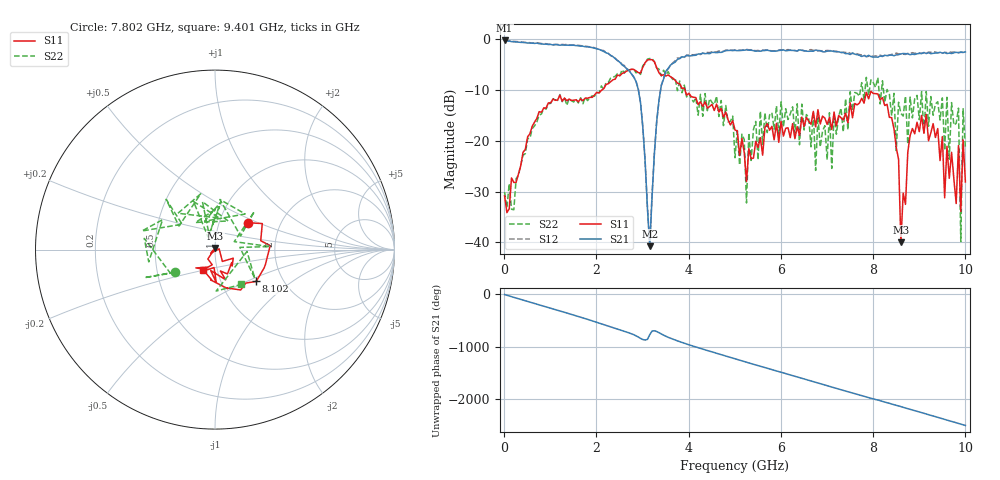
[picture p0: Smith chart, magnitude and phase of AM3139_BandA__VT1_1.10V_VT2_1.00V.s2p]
! Date/Time: Tue, Nov 13, 2018 4:56 PM
! Network Analyzer: Agilent Technologies E8364B Rev: A.07.50.67
! Sweep from 0.010 to 10.000 GHz, 201 Points, Sweep Type: LIN
! Power Supply: 1.100 V, 0.000 A
# Hz S DB R 50
!freq MagS11 AngS11 MagS21 AngS21 MagS12 AngS12 MagS22 AngS22
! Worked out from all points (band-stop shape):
!   201 points, 10 MHz to 10 GHz, reference 50 ohm
!   highest |S21| = -0.21 dB at 10 MHz (marker M1); lowest = -40.8 dB at 3.157 GHz (marker M2)
!   |S21| within 3 dB of the highest: start of sweep to 2.32 GHz; 4.069 GHz to 7.72 GHz (3.65 GHz wide, 61.9 % of centre)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
!   lowest |S11| = -40.0 dB at 8.601 GHz (marker M3), VSWR 1.02, Z = 50.2 + j0.98 ohm
!   |S11| at or under -10 dB: start of sweep to 2.116 GHz; 3.921 GHz to end of sweep
!   |S22| runs from -39.9 to -3.8 dB; largest |S21 - S12| = 0.03
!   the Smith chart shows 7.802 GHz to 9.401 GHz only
!   S11 on the Smith chart (normalised r, x): 7.802 GHz: 1.36, +0.43; 8.102 GHz: 1.47, -0.57; 9.401 GHz: 0.85, -0.20
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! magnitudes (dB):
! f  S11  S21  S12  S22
! 10 MHz  -30.9  -0.2  -0.2  -30.1
! 1.708 GHz  -12.1  -1.3  -1.3  -12.7
! 2.857 GHz  -6.2  -8.2  -8.2  -6.6
! 3.157 GHz  -4.0  -40.8  -40.5  -3.8
! 3.357 GHz  -6.6  -12.0  -12.1  -5.9
! 5.005 GHz  -17.9  -2.2  -2.0  -23.3
! 5.255 GHz  -28.0  -2.0  -2.0  -32.2
! 5.554 GHz  -19.4  -2.3  -2.3  -14.2
! 6.703 GHz  -14.2  -2.3  -2.2  -14.2
! 7.103 GHz  -17.8  -2.3  -2.2  -25.4
! 7.802 GHz  -12.6  -3.2  -3.0  -11.9
! 8.102 GHz  -10.7  -3.5  -3.3  -7.5
! 8.352 GHz  -15.4  -3.1  -3.1  -10.8
! 8.551 GHz  -23.7  -3.0  -2.8  -12.4
! 8.601 GHz  -40.0  -2.9  -2.9  -14.6
! 8.851 GHz  -17.6  -2.9  -2.6  -15.5
! 9.401 GHz  -17.6  -2.7  -2.6  -12.3
! 9.55 GHz  -31.2  -2.6  -2.5  -21.9
! 9.85 GHz  -20.9  -2.6  -2.6  -13.5
! 9.9 GHz  -33.9  -2.5  -2.6  -39.9
! 9.95 GHz  -19.8  -2.6  -2.5  -13.7
! 10 GHz  -28.1  -2.5  -2.4  -21.3
